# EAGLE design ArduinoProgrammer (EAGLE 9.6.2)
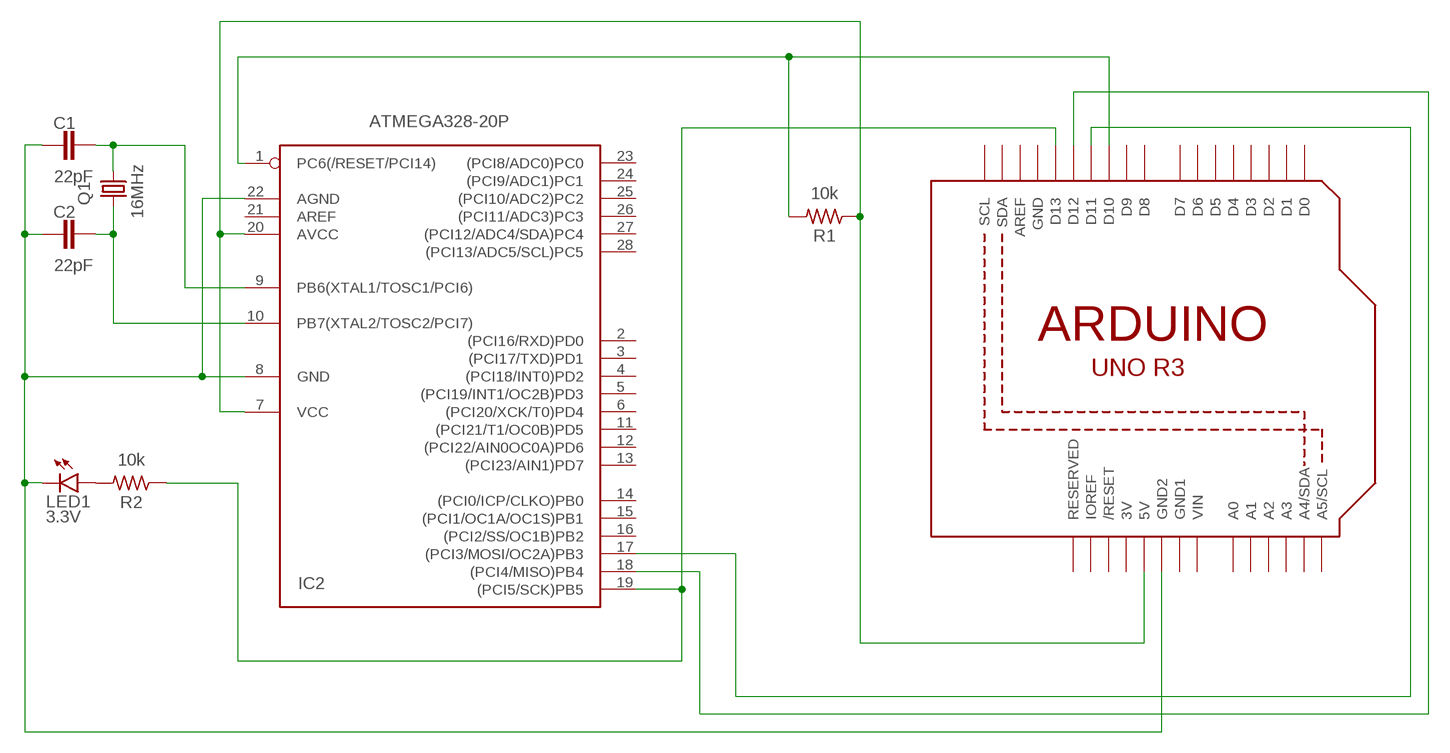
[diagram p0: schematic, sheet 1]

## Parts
C1  22pF  C-EU025-024X044  [C025-024X044]
C2  22pF  C-EU025-024X044  [C025-024X044]
IC2  ATMEGA328-20P  [DIL28-3]
LED1  3.3V  LED3MM  [LED3MM]
Q1  16MHz  CRYSTALHC33U-V  [HC33U-V]
R1  10k  R-US_AXIAL-11.7MM-PITCH  [RESAD1176W63L850D250B]
R2  10k  R-US_AXIAL-11.7MM-PITCH  [RESAD1176W63L850D250B]
U1  ARDUINOR3-DIMENSION  [ARDUINOR3]

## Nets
N$2: IC2.17((PCI3/MOSI/OC2A)PB3) U1.D11
N$3: IC2.18((PCI4/MISO)PB4) U1.D12
N$4: IC2.19((PCI5/SCK)PB5) R2.1 U1.D13
N$5: C1.1 C2.1 IC2.8(GND) IC2.22(AGND) LED1.K(C) U1.GND2
N$6: IC2.7(VCC) IC2.20(AVCC) R1.1 U1.5V
N$7: C1.2 IC2.9(PB6(XTAL1/TOSC1/PCI6)) Q1.1
N$8: C2.2 IC2.10(PB7(XTAL2/TOSC2/PCI7)) Q1.2
N$9: IC2.1(PC6(/RESET/PCI14)) R1.2 U1.D10
N$10: LED1.A R2.2
Unconnected: IC2.2((PCI16/RXD)PD0) IC2.3((PCI17/TXD)PD1) IC2.4((PCI18/INT0)PD2) IC2.5((PCI19/INT1/OC2B)PD3) IC2.6((PCI20/XCK/T0)PD4) IC2.11((PCI21/T1/OC0B)PD5) IC2.12((PCI22/AIN0OC0A)PD6) IC2.13((PCI23/AIN1)PD7) IC2.14((PCI0/ICP/CLKO)PB0) IC2.15((PCI1/OC1A/OC1S)PB1) IC2.16((PCI2/SS/OC1B)PB2) IC2.21(AREF) IC2.23((PCI8/ADC0)PC0) IC2.24((PCI9/ADC1)PC1) IC2.25((PCI10/ADC2)PC2) IC2.26((PCI11/ADC3)PC3) IC2.27((PCI12/ADC4/SDA)PC4) IC2.28((PCI13/ADC5/SCL)PC5) U1.A0 U1.A1 U1.A2 U1.A3 U1.A4(A4/SDA) U1.A5(A5/SCL) U1.AREF U1.D0 U1.D1 U1.D2 U1.D3 U1.D4 U1.D5 U1.D6 U1.D7 U1.D8 U1.D9 U1.IOREF U1.RESERVED U1.RESET(/RESET) U1.SCL U1.SDA

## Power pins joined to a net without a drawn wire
3V: U1.3V
GND: U1.GND
GND1: U1.GND1
VIN: U1.VIN

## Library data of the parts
C1 C2 = rcl:C-EU: CAPACITOR, European symbol; SPICEPREFIX: C
IC2 = atmega328:ATMEGA328*P: MICROCONTROLLER 32 kBytes FLASH 2 kBytes SRAM 1 kBytes EEPROM USART 8-channel 10 bit ADC
LED1 = led:LED: LED
Q1 = crystal:CRYSTAL: CRYSTAL; OC_FARNELL: unknown; OC_NEWARK: unknown
R1 R2 = Resistor:R-US: Resistor Fixed - ANSI; CATEGORY: Resistor; SUB-CATEGORY: Fixed
U1 = adafruit:ARDUINOR3: This is a new object for the new Arduino R3 - with extra pins that you may want to use (such as IOref, and duplicated A4/A5

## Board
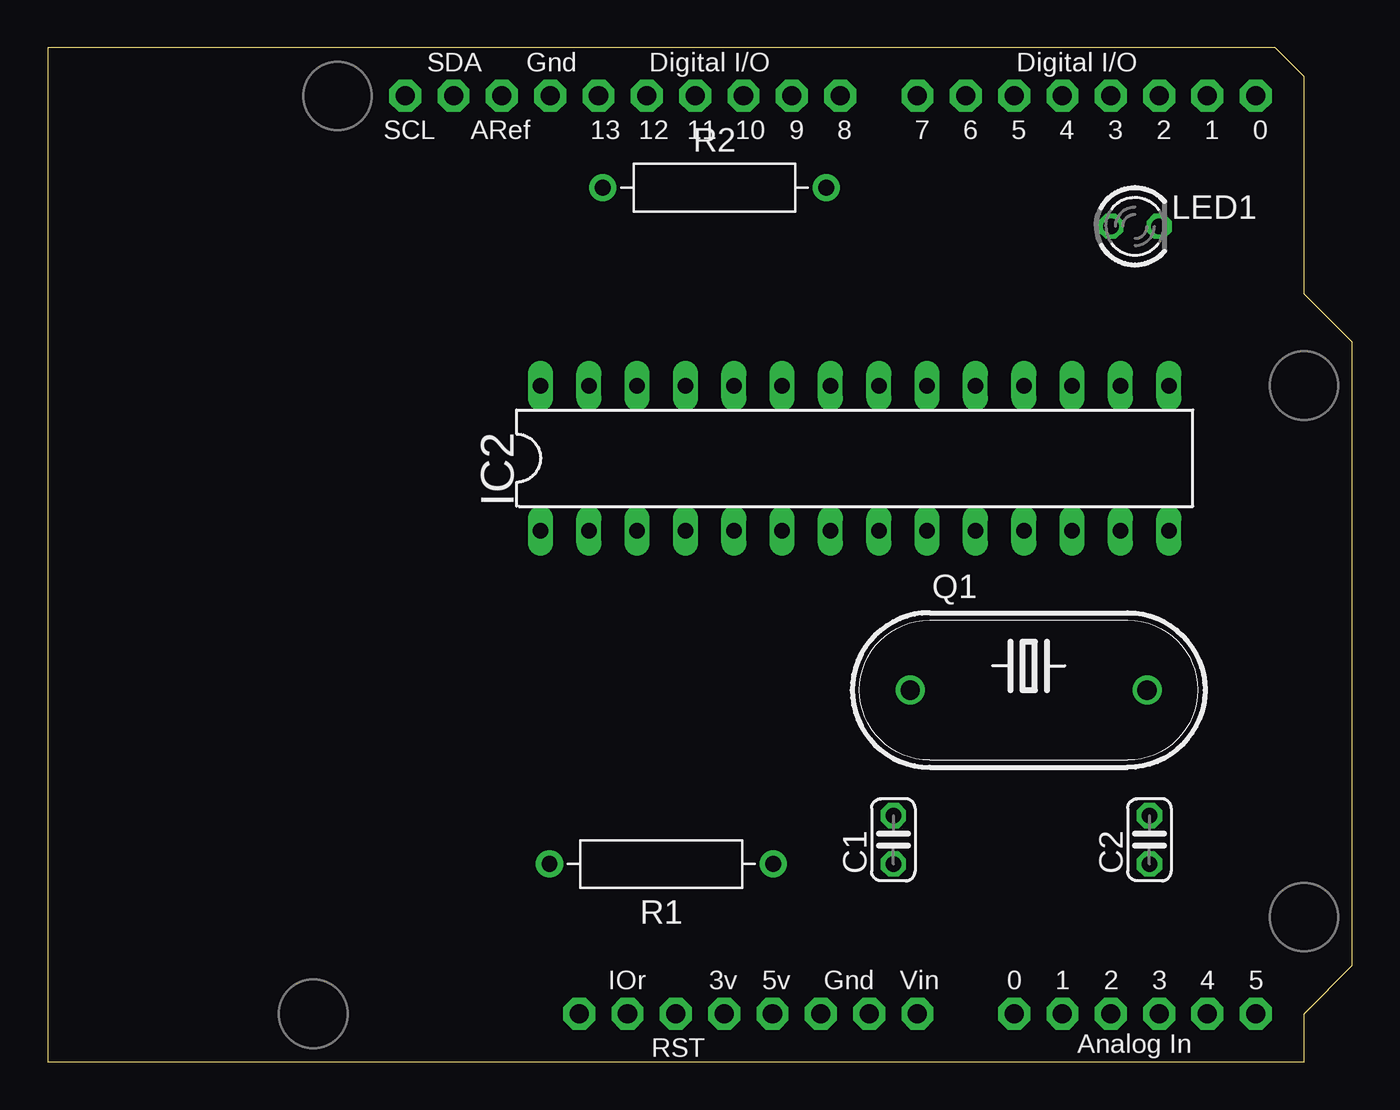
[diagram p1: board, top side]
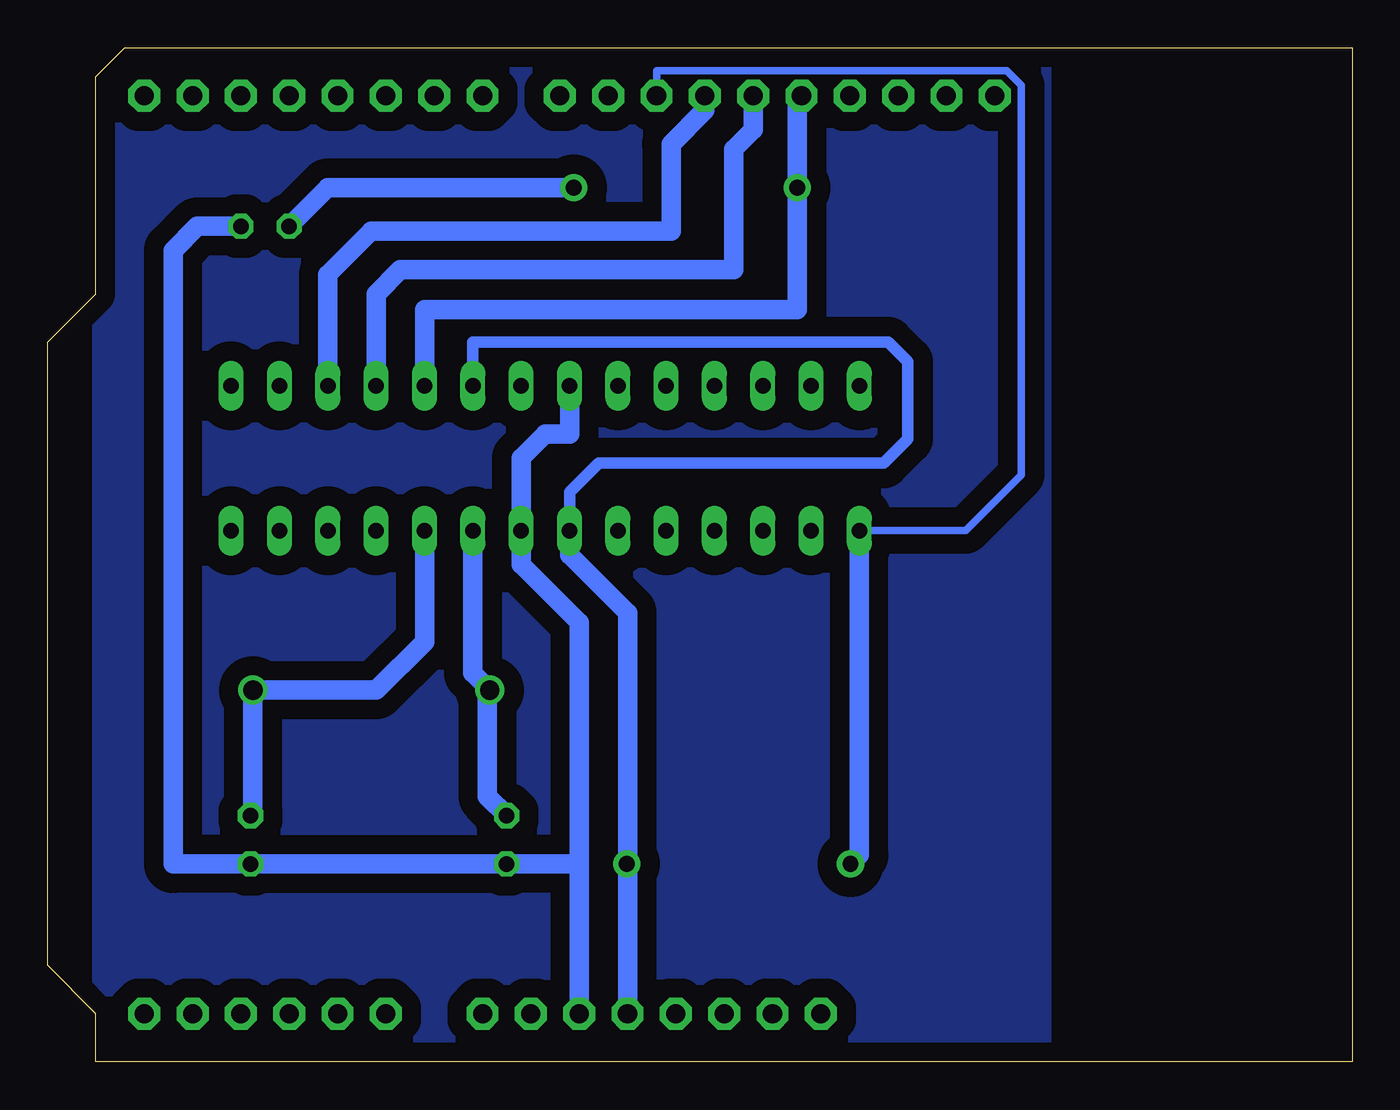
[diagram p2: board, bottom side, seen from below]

Size 68.58 x 53.34 mm. Coordinates in mm from the lower left corner, seen from the top.
Copper layers (1*16): Top 0.035mm / dielectric 1.5mm / Bottom 0.035mm
Design rules "default": minimum track width 6mil, minimum drill 0.35mm, track to track 6mil, track to pad 6mil, pad to pad 6mil, via to via 6mil, smd to smd 6mil, copper to edge 40mil, drill to drill 6mil, minimum pad ring 10mil, minimum via ring 8mil, stop-mask expansion 4mil, vias tented up to drill 0mil, thermal gap 10mil

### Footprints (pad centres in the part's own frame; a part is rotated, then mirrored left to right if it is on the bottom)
C025-024X044 = drill 0.813 octagon: 1 -1.27,0; 2 1.27,0
DIL28-3 = drill 0.813 long: 1 -16.51,-3.81; 2 -13.97,-3.81; 3 -11.43,-3.81; 4 -8.89,-3.81; 5 -6.35,-3.81; 6 -3.81,-3.81; 7 -1.27,-3.81; 8 1.27,-3.81; 9 3.81,-3.81; 10 6.35,-3.81; 11 8.89,-3.81; 12 11.43,-3.81; 13 13.97,-3.81; 14 16.51,-3.81; 15 16.51,3.81; 16 13.97,3.81; 17 11.43,3.81; 18 8.89,3.81; 19 6.35,3.81; 20 3.81,3.81; 21 1.27,3.81; 22 -1.27,3.81; 23 -3.81,3.81; 24 -6.35,3.81; 25 -8.89,3.81; 26 -11.43,3.81; 27 -13.97,3.81; 28 -16.51,3.81
LED3MM = drill 0.813 octagon: A -1.27,0; K 1.27,0
HC33U-V = drill 1.016: 1 -6.223,0; 2 6.223,0
RESAD1176W63L850D250B = drill 0.83 pad 1.43: 1 -5.88,0; 2 5.88,0
ARDUINOR3 = drill 1 pad 1.676 octagon: 3V 35.56,2.54; 5V 38.1,2.54; A0 50.8,2.54; A1 53.34,2.54; A2 55.88,2.54; A3 58.42,2.54; A4 60.96,2.54; A5 63.5,2.54; AREF 23.876,50.8; D0 63.5,50.8; D1 60.96,50.8; D2 58.42,50.8; D3 55.88,50.8; D4 53.34,50.8; D5 50.8,50.8; D6 48.26,50.8; D7 45.72,50.8; D8 41.656,50.8; D9 39.116,50.8; D10 36.576,50.8; D11 34.036,50.8; D12 31.496,50.8; D13 28.956,50.8; GND 26.416,50.8; GND1 43.18,2.54; GND2 40.64,2.54; IOREF 30.48,2.54; RESERVED 27.94,2.54; RESET 33.02,2.54; SCL 18.796,50.8; SDA 21.336,50.8; VIN 45.72,2.54

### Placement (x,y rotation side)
C1  44.45,11.68 90 top
C2  57.91,11.68 90 top
IC2  42.42,31.75 0 top
LED1  57.15,43.94 0 top
Q1  51.56,19.56 0 top
R1  32.26,10.41 180 top
R2  35.05,45.97 0 top
U1  0,0 0 top

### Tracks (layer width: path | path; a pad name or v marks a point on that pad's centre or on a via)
N$1
  pour Bottom (isolate 1.016): 16,53.34 16,0 66.04,0 66.04,51.82 64.52,53.34 16.26,53.34
N$2
  Bottom 1.016: U1.D11 34.04,50.04 35.81,48.26 35.81,43.69 51.56,43.69 53.85,41.4 IC2.17
N$3
  Bottom 1.016: U1.D12 31.5,49.02 32.51,48.01 32.51,41.66 50.04,41.66 51.31,40.39 IC2.18
N$4
  Bottom 0.152: U1.D13 29.17,50.58
  Bottom 1.016: IC2.19 48.77,39.57 29.17,39.57 R2.1 29.17,50.58
N$5
  Bottom 0.152: U1.GND2 40.64,10.41
  Bottom 1.016: U1.GND2 40.64,23.11 43.69,26.16 IC2.8 43.69,31.75 42.42,33.02 41.15,33.02 IC2.22 | 40.64,10.41 C1.1 C2.1 61.98,10.41 61.98,42.67 60.71,43.94 LED1.K
N$6
  Bottom 0.152: U1.5V 38.1,10.92 | 38.1,10.38 R1.1
  Bottom 0.61: IC2.20 46.23,37.85 24.38,37.85 23.37,36.83 23.37,32.77 24.64,31.5 39.62,31.5 41.15,29.97 IC2.7
  Bottom 1.016: IC2.7 41.15,26.67 38.1,23.62 38.1,10.92 | U1.5V 38.1,10.38
N$7
  Bottom 1.016: IC2.9 46.23,20.45 Q1.1 45.47,19.43 45.47,13.97 C1.2
N$8
  Bottom 1.016: C2.2 57.78,13.08 Q1.2 51.31,19.56 48.77,22.1 IC2.10
N$9
  Bottom 0.406: IC2.1 20.32,27.94 17.4,30.86 17.4,51.36 18.16,52.12 36.58,52.12 U1.D10
  Bottom 1.016: IC2.1 25.91,10.88 R1.2
N$10
  Bottom 1.016: R2.2 53.85,45.97 LED1.A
